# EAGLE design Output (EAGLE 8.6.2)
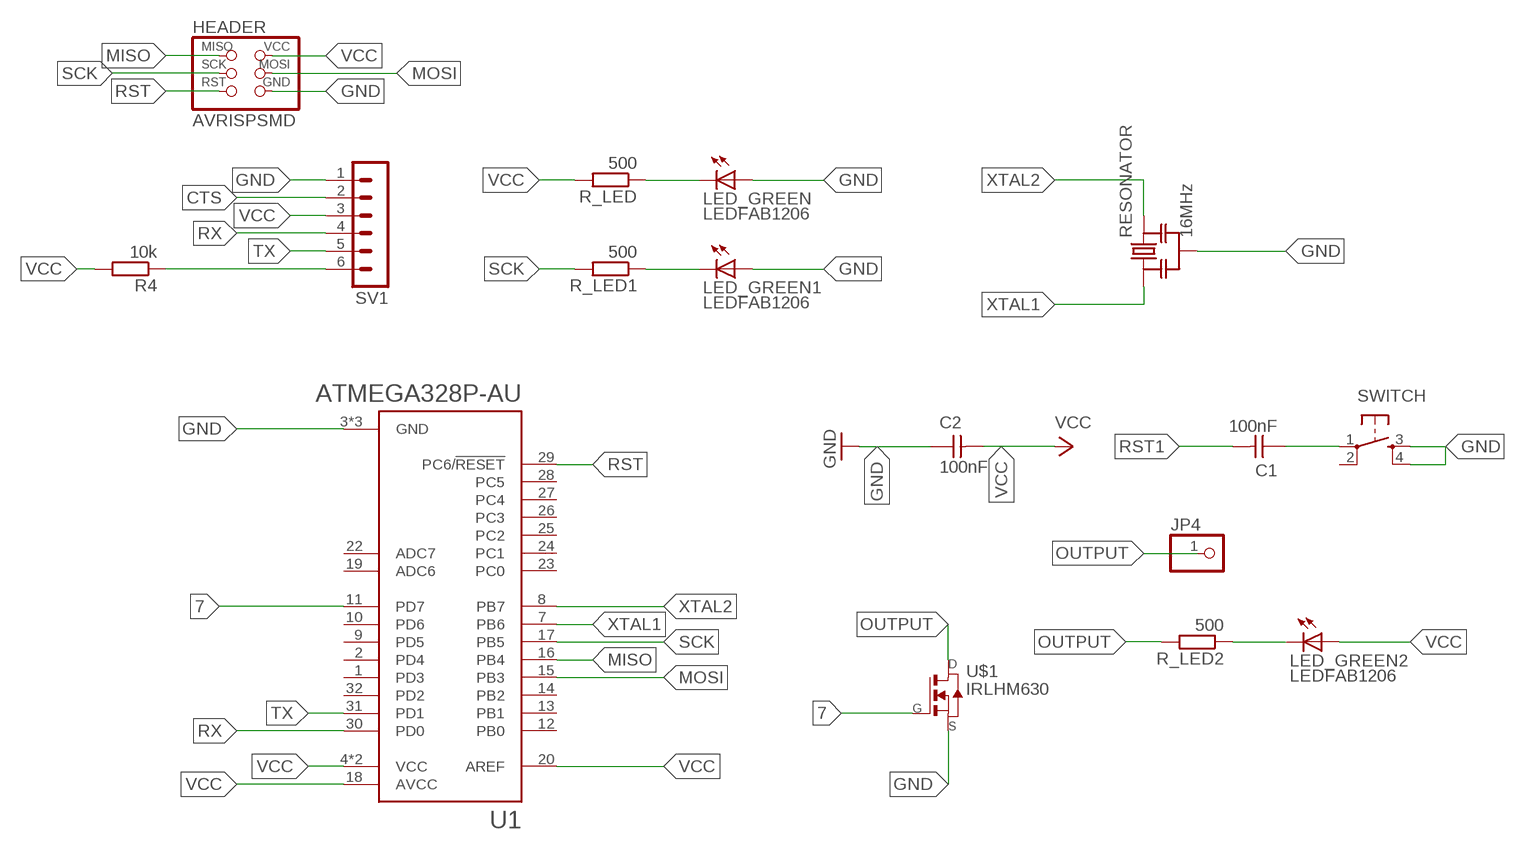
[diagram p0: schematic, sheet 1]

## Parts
C1  100nF  CAP-UNPOLARIZEDFAB  [C1206FAB]
C2  100nF  CAP-UNPOLARIZEDFAB  [C1206FAB]
HEADER  AVRISPSMD  [2X03SMD]
JP4  PINHD-1X1  [1X01]
LED_GREEN  LEDFAB1206  [LED1206FAB]
LED_GREEN1  LEDFAB1206  [LED1206FAB]
LED_GREEN2  LEDFAB1206  [LED1206FAB]
R4  10k  R-EU_R1206  [R1206]
R_LED  500  R-EU_R1206  [R1206]
R_LED1  500  R-EU_R1206  [R1206]
R_LED2  500  R-EU_R1206  [R1206]
RESONATOR  16MHz  RESONATOR-MURATACSTCR_G  [RESONATOR_MURATA3]
SV1  MA06-1  [MA06-1]
SWITCH  6MM_SWITCH6MM_SWITCH  [6MM_SWITCH]
U1  ATMEGA328P-AU  [QFP80P900X900X120-32N]
U$1  IRLHM630  [IRF-PQFN3.3X3.3B]

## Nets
7: U1.11(PD7) U$1.G
CTS: SV1.2
GND: C2.1 HEADER.6(GND) LED_GREEN1.1(A) LED_GREEN.1(A) RESONATOR.2 SV1.1 SWITCH.3(S) SWITCH.4(S1) U1.3(GND) U1.5(GND) U1.21(GND) U$1.S
MISO: HEADER.1(MISO) U1.16(PB4)
MOSI: HEADER.4(MOSI) U1.15(PB3)
N$1: LED_GREEN1.2(C) R_LED1.1
N$2: LED_GREEN2.2(C) R_LED2.1
N$21: LED_GREEN.2(C) R_LED.1
OUTPUT: JP4.1 R_LED2.2 U$1.D
RST: C1.1 HEADER.5(RST) SWITCH.1(P) U1.29(PC6/!RESET)
RST1: C1.2 R4.1 SV1.6
RX: SV1.4 U1.30(PD0)
SCK: HEADER.3(SCK) R_LED1.2 U1.17(PB5)
TX: SV1.5 U1.31(PD1)
VCC: C2.2 HEADER.2(VCC) LED_GREEN2.1(A) R4.2 R_LED.2 SV1.3 U1.4(VCC) U1.6(VCC) U1.18(AVCC) U1.20(AREF)
XTAL1: RESONATOR.1 U1.7(PB6)
XTAL2: RESONATOR.3 U1.8(PB7)
Unconnected: SWITCH.2(P1) U1.1(PD3) U1.2(PD4) U1.9(PD5) U1.10(PD6) U1.12(PB0) U1.13(PB1) U1.14(PB2) U1.19(ADC6) U1.22(ADC7) U1.23(PC0) U1.24(PC1) U1.25(PC2) U1.26(PC3) U1.27(PC4) U1.28(PC5) U1.32(PD2)

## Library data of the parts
C1 C2 = fab:CAP-UNPOLARIZED
HEADER = fab:AVRISP
JP4 = pinhead:PINHD-1X1: PIN HEADER
LED_GREEN LED_GREEN1 LED_GREEN2 = fab:LED: LED
R4 R_LED R_LED1 R_LED2 = resistor:R-EU_: RESISTOR, European symbol
RESONATOR = m-pad-2.1:RESONATOR-MURATA: Murata ceramic Resonator "ceralock" CSTCE series with built in load capacitance +- 0.5% tolerance 12.51MHz to 19.99MHz 16MHz murata part#: CSTCE16M0V53-R0 16MHz digikey part#: 490-1198-1-ND $1.33 each
SV1 = con-lstb:MA06-1: PIN HEADER; OC_FARNELL: unknown; OC_NEWARK: unknown
SWITCH = fab:6MM_SWITCH: OMRON SWITCH
U1 = ATMEGA328P-AU:ATMEGA328P-AU: ATmega Series 20 MHz 32 KB Flash 2 KB SRAM 8-Bit Microcontroller - TQFP-32; AVAILABILITY: Good; DESCRIPTION: ATmega Series 20 MHz 32 KB Flash 2 KB SRAM 8-Bit Microcontroller - TQFP-32; MF: Atmel; MP: ATMEGA328P-AU; PACKAGE: TQFP-32 Atmel; PRICE: 2.38 USD
U$1 = fab:IRLHM630

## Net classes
0 default: clearance 0.205 mm

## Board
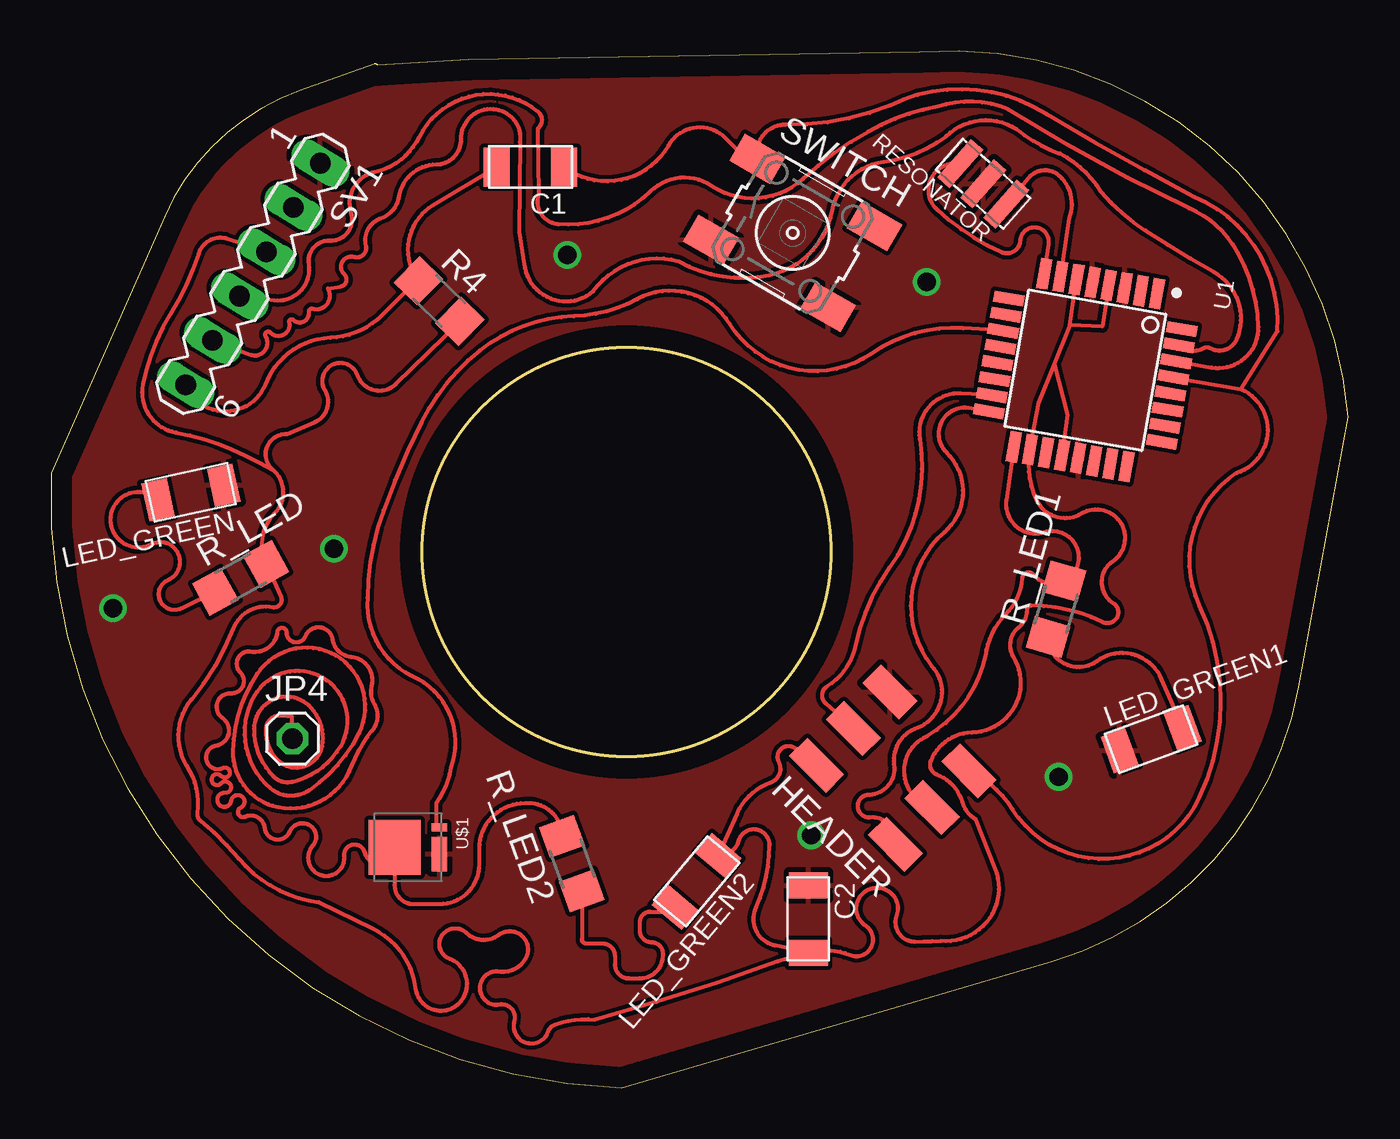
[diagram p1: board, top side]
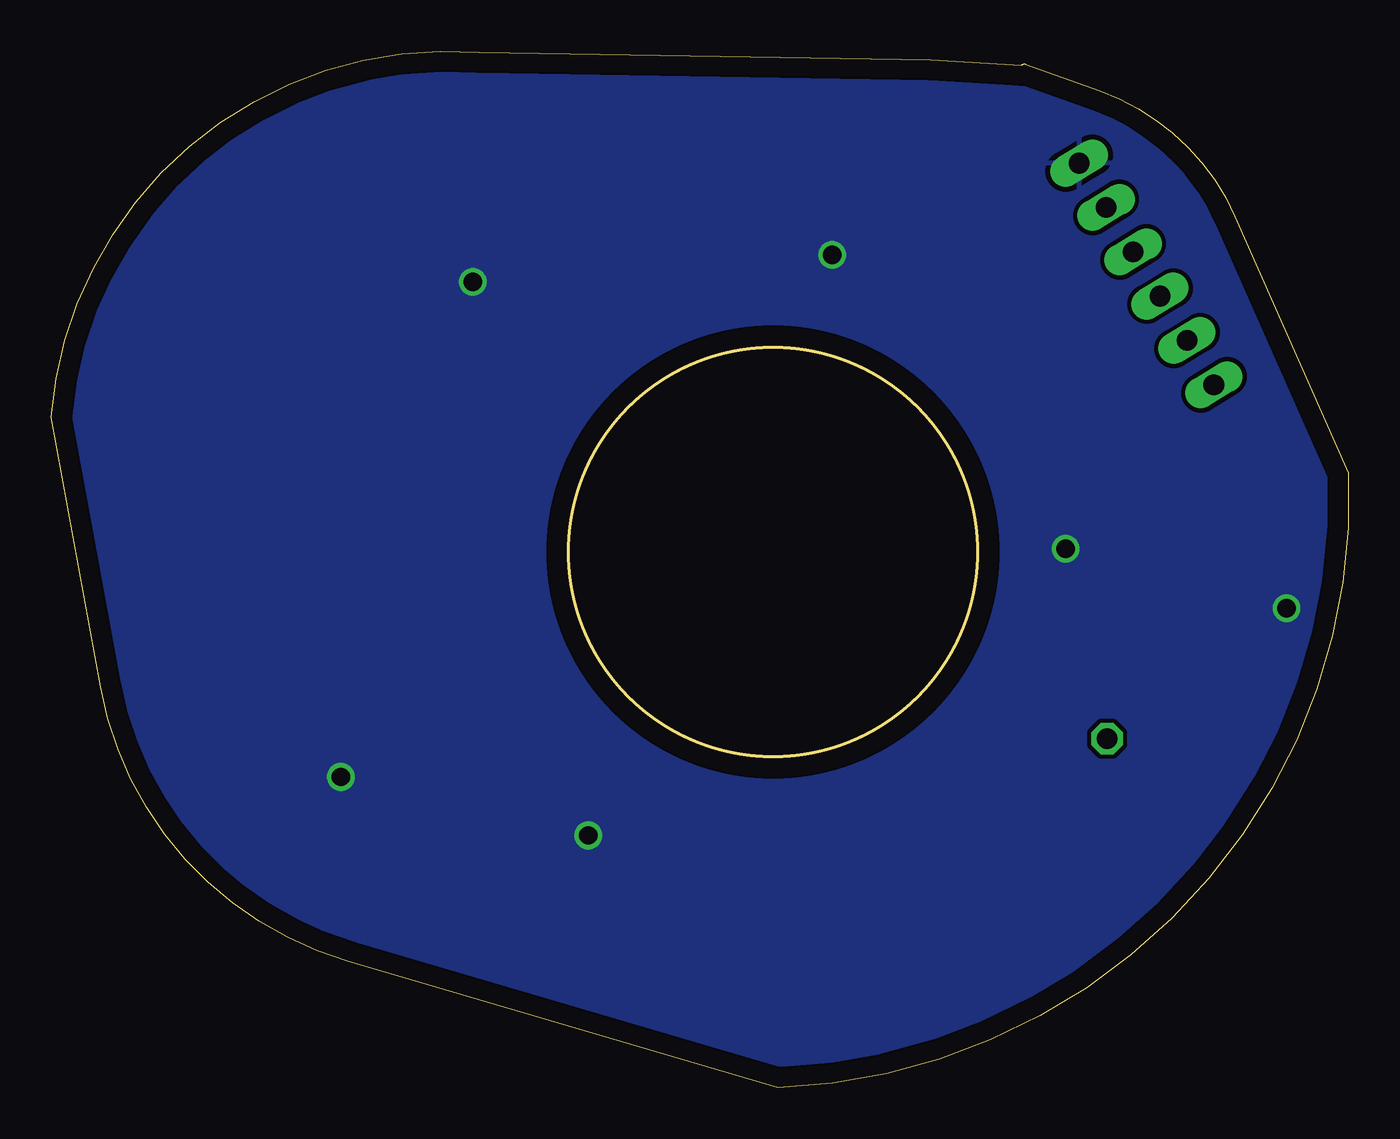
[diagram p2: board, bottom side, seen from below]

Size 63.52 x 50.75 mm. Coordinates in mm from the lower left corner, seen from the top.
Outline: 16,50.07 arc65 15.81,50.11 12.16,48.8 arc46 5.56,42.65 0,30.09 arc90 27.94,0 49,6.18 arc63 61.1,19.61 63.52,32.82 arc90 42.53,50.7 20.45,50.32 16,50.07
Outline: circle at 28.17,26.22 radius 10
Copper layers (1*16): Top 0.035mm / dielectric 1.5mm / Bottom 0.035mm
Design rules "default *": minimum track width 6mil, minimum drill 0.35mm, track to track 8mil, track to pad 8mil, pad to pad 8mil, via to via 8mil, smd to smd 8mil, copper to edge 40mil, drill to drill 8mil, minimum pad ring 10mil, minimum via ring 8mil, stop-mask expansion 4mil, vias tented up to drill 0mil, thermal gap 10mil

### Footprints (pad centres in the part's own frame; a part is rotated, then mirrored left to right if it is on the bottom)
C1206FAB = smd 1.27 x 1.905: 1 -1.651,0; 2 1.651,0
2X03SMD = smd 2.54 x 1.27: 1 -2.54,2.54; 2 2.92,2.54; 3 -2.54,0; 4 2.92,0; 5 -2.54,-2.54; 6 2.92,-2.54
1X01 = drill 1.016 octagon: 1 0,0
LED1206FAB = smd 1.27 x 1.905: 1 -1.651,0; 2 1.651,0
R1206 = smd 1.6 x 1.803: 1 -1.422,0; 2 1.422,0
RESONATOR_MURATA3 = smd 0.8 x 2.5: 1 -1.5,0; 2 0,0; 3 1.5,0
MA06-1 = drill 1.016 long: 1 -6.35,0; 2 -3.81,0; 3 -1.27,0; 4 1.27,0; 5 3.81,0; 6 6.35,0
6MM_SWITCH = smd 2.286 x 1.524: 1 -3.302,2.286; 2 3.302,2.286; 3 -3.302,-2.286; 4 3.302,-2.286
QFP80P900X900X120-32N = smd 1.5 x 0.55: 1 -4.3,2.8; 2 -4.3,2; 3 -4.3,1.2; 4 -4.3,0.4; 5 -4.3,-0.4; 6 -4.3,-1.2; 7 -4.3,-2; 8 -4.3,-2.8; 17 4.3,-2.8; 18 4.3,-2; 19 4.3,-1.2; 20 4.3,-0.4; 21 4.3,0.4; 22 4.3,1.2; 23 4.3,2; 24 4.3,2.8 | smd 0.55 x 1.5: 9 -2.8,-4.3; 10 -2,-4.3; 11 -1.2,-4.3; 12 -0.4,-4.3; 13 0.4,-4.3; 14 1.2,-4.3; 15 2,-4.3; 16 2.8,-4.3; 25 2.8,4.3; 26 2,4.3; 27 1.2,4.3; 28 0.4,4.3; 29 -0.4,4.3; 30 -1.2,4.3; 31 -2,4.3; 32 -2.8,4.3
IRF-PQFN3.3X3.3B = smd 2.7 x 2.54: D 0,-1.27 | smd 0.39 x 0.77: G -0.975,0.925 | smd 1.69 x 0.77: S 0.325,0.925

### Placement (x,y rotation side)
C1  23.47,45.07 180 top
C2  37.08,8.25 270 top
HEADER  41.35,15.51 135 top
JP4  11.82,17.08 0 top
LED_GREEN  6.85,29.14 192.4 top
LED_GREEN1  53.86,17.06 20 top
LED_GREEN2  31.61,10.09 230 top
R4  19,38.51 315.6 top
R_LED  9.28,24.96 28.9 top
R_LED1  49.21,23.43 74 top
R_LED2  25.5,10.96 110 top
RESONATOR  45.64,44.25 138.6 top
SV1  9.89,39.84 238.7 top
SWITCH  36.31,41.85 330 top
U1  50.64,35.13 260 top
U$1  18.09,11.76 270 top

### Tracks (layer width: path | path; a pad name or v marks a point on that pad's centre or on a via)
7
  Top 0.2: U1.11 44.66,37.18 arc38 40.16,35.93 arc-93 33.23,37.39 arc87 28.7,38.61 arc-26 25.59,37.77 arc36 21,36.09 arc25 18.14,32.58 arc6 16.28,28.26 arc20 15.5,23.98 arc69 17.67,20.16 arc-86 19.57,15.65 arc-26 18.85,13.91 18.85,12.74 U$1.G
GND  (via drill 0.9)
  other vias: 13.86,26.39 49.34,15.21 37.23,12.35 42.87,39.44 25.27,40.78 3.03,23.46
  pour Top: -37.68,78.67 -0.24,-8.88 7.37,-16.26 75.76,-78.44 85.51,-52.14 85.51,79.94 75.35,90.1 -26.25,90.1
  pour Bottom: -11.95,28.08 1.62,41.65 1.62,52.26 8.59,59.22 28.17,59.22 51.51,59.22 62.64,48.09 67.98,42.75 67.98,26.02 67.98,11.04 53.51,-3.43 17.72,-3.43 15.19,-0.9 -4.71,19 -8.78,19 -8.78,24.7 -12,27.92
MISO
  Top 0.2: U1.16 44.93,33.27 arc145 43.84,31.1 arc-95 43.74,27.19 arc87 43.12,20.64 arc-111 42.43,17.62 arc84 41.29,15.67 arc-93 39.96,14.33 arc177 40.09,13.24 arc-103 HEADER.1
MOSI
  Top 0.2: U1.15 44.54,33.99 arc102 42.53,31.76 arc-44 41.06,25.47 arc24 39.39,21.64 arc-46 37.99,19.63 arc106 37.91,18.82 arc0 HEADER.4
N$1
  Top 0.2: LED_GREEN1.2 54.37,20.01 arc102 51.19,20.87 arc-125 R_LED1.1
N$2
  Top 0.2: R_LED2.1 25.99,7.26 arc90 26.2,7.06 27,7.06 arc-90 27.6,6.45 27.6,6.03 arc90 28.28,5.35 28.83,5.35 arc90 29.96,6.48 29.96,6.55 arc90 29.41,7.11 | 29.41,7.11 | 29.41,7.11 arc-90 28.83,7.68 28.83,8.11 arc-90 29.34,8.61 30.33,8.61 arc90 LED_GREEN2.2
N$21
  Top 0.2: R_LED.1 6.39,23.46 arc-182 5.74,24.86 arc184 4.91,26.59 arc-252 LED_GREEN.2
OUTPUT
  Top 0.2: JP4.1 11.8,18.16 11.25,18.21 arc90 10.53,17.61 arc51 11.1,16.03 arc124 13.27,16.71 arc59 12.6,18.73 arc131 9.93,17.56 arc46 10.89,15.23 arc57 11.8,14.97 arc47 14.18,16.71 arc180 9.96,19.19 arc80 10.74,14.66 arc74 12.63,14.56 arc30 15.08,17.35 arc173 10.09,20.25 arc32 8.9,16.5 arc81 11.12,13.73 arc80 14.72,15.75 arc-19 15.73,17.48 arc71 15.84,18.78 arc-45 15.71,19.66 arc99 14.7,21.08 arc-76 13.79,21.93 arc150 12.44,22.09 arc-159 11.54,22.27 arc175 11.07,22.3 arc-42 10.74,21.62 arc-52 9.78,21.34 arc144 9.26,20.33 arc-138 8.8,19.29 arc149 8.38,18.1 arc-136 8.07,16.73 arc196 8.41,15.65 arc-253 8.33,15.26 arc275 8.33,14.89 arc-233 8.51,14.43 arc268 8.82,14.04 arc-237 9.29,13.7 arc179 9.49,13.26 arc-108 10.45,12.72 arc151 11.69,12.54 arc-198 12.81,11.84 arc228 14.36,11.35 arc-172 15.34,11.53 arc169 U$1.D 16.82,9.9 arc90 17.73,8.99 19.04,8.99 arc90 20.97,10.92 20.97,11.7 arc-90 23.21,13.93 23.38,13.93 arc-90 R_LED2.2
RST
  Top 0.2: 58.25,34.21 arc-138 58.04,30.09 arc82 56.21,23.64 arc-50 56.21,14.18 arc-123 47.08,13.63 arc33 HEADER.5 | U1.29 58.25,34.21 | 58.25,34.21 60.05,37.03 arc71 55.98,43.61 arc-3 48.76,47.65 arc58 41.06,48.09 arc-23 35.95,47.14 arc104 SWITCH.1 34.03,45.48 33.02,46.49 arc105 30.22,46.12 arc-97 C1.1
RST1
  Top 0.2: C1.2 18.7,43.2 arc96 R4.1 17.89,39.51 16.21,37.83 arc-43 13.67,36.71 arc66 10.5,34.44 arc-137 SV1.6
RX
  Top 0.2: SV1.4 10.94,38.55 arc106 12.63,40.31 arc-102 13.66,41.48 arc110 14.7,42.82 arc-95 15.86,44.84 arc51 18.04,46.55 arc-103 23.83,47.79 arc-101 23.83,46.96 23.89,43.72 arc104 24.83,42.27 arc49 29.35,43.88 arc-78 32.35,44.15 arc77 36.82,44.5 arc-14 40.02,46.81 arc-18 43.41,48.03 arc-40 46.86,47.91 arc7 55.73,43.05 arc-33 57.83,41.32 arc-33 59.12,37.24 arc-101 56.82,35.26 U1.30
SCK
  Top 0.2: U1.17 46.77,28.76 arc116 48.62,27.19 arc-171 R_LED1.2 arc-77 48.1,25.11 arc136 47.55,24.93 arc-41 46.74,23.17 arc38 45.75,21.16 arc-48 42.89,17.2 arc142 HEADER.3
TX
  Top 0.2: SV1.5 9.75,35.89 arc142 10.5,36.79 arc-167 10.74,36.97 arc149 11.67,37.49 arc-148 11.85,37.59 arc142 12.63,37.98 arc-114 12.81,38.14 arc138 13.56,39.12 14.18,39.22 arc127 14.36,39.82 arc-153 14.85,40.67 arc120 15.42,41.22 arc-84 16.15,42.56 arc61 17.05,43.65 arc-81 18.86,45.2 arc91 20.08,46.44 arc-129 22.44,47.61 arc-60 22.96,46.31 22.92,41.92 23.17,40.31 arc124 26.54,38.99 arc-70 30.73,40.46 arc41 35.16,39.78 arc68 38.25,42.94 arc-72 40.78,45.33 arc29 43.83,46.59 arc-77 47.28,46.92 arc21 49.4,45.74 arc-31 51.4,43.87 arc16 53.58,41.96 arc4 56.91,39.95 arc-84 58.03,36.62 arc-96 56.76,36.2 arc60 56.42,36.2 arc-74 U1.31
VCC
  Top 0.2: 49.11,35.39 48.36,33.54 U1.18 arc36 48.25,28.78 arc96 50.46,28.11 arc-177 51.97,25.76 arc114 52,23.73 arc-174 51.48,22.79 arc26 48,23.6 arc90 47.78,23.38 arc-51 47.37,22.52 arc82 47.11,21.08 arc-120 45.08,17.38 arc67 43.07,16 arc91 43.36,15.33 arc-53 44.62,13.97 arc43 45.26,13.14 46.22,10.7 arc-117 43.56,7.18 arc-4 42.29,7.15 arc-110 41.4,8.43 arc256 39.88,7.92 arc-169 39.13,6.49 arc38 C2.2 | 49.11,35.39 49.89,37.3 49.89,37.32 | 49.89,37.32 U1.6 | U1.4 51.47,37.27 49.89,37.32 | 49.11,35.39 49.77,32.93 U1.20 | 10.87,30.24 arc-94 10.97,28.15 arc68 R_LED.2 11.25,24.03 arc-126 10.84,23.51 arc80 8.92,22.48 arc-18 6.85,18.98 arc72 6.65,15.75 arc-39 7.16,13.45 arc58 7.32,13.06 arc-10 9.18,11.22 arc42 13.12,9.07 15.75,7.78 arc-57 17.84,4.87 arc128 19.99,4.14 arc114 19.52,6.3 arc-203 20.32,7.58 arc80 21.93,7.48 arc-152 23.26,6.38 arc-73 21.93,5.67 arc199 21.95,4.07 arc-116 22.68,3.26 arc176 24.34,2.74 arc-51 24.69,3.09 arc-25 26.63,3.33 arc5 35.58,6.17 C2.2 | 10.87,30.24 arc-143 11.56,32 12.93,32.59 arc104 13.35,34.23 arc-185 15.01,34.88 arc115 16.87,34.44 R4.2 | SV1.3 8.64,41.55 arc91 7.22,40.83 arc-14 5.84,37.85 arc21 4.5,34.41 arc91 6.1,32.08 arc-14 8.82,31.25 arc-5 10.87,30.24 | LED_GREEN2.1 | LED_GREEN2.1 33.6,13.43 arc-47 35.23,14.93 arc98 35.64,15.95 arc-189 36.6,16.37 arc75 HEADER.2 | C2.2 35.44,6.95 arc-102 34.52,8.8 arc24 35.18,11.87 arc165 33.66,12.07 arc-79 LED_GREEN2.1
XTAL1
  Top 0.2: RESONATOR.1 47.88,44.56 arc-93 49.37,44.65 arc-69 49.84,42.55 U1.7
XTAL2
  Top 0.2: U1.8 48.85,41.31 arc185 47.44,41.45 arc-110 46.54,40.9 arc-19 43.39,42.98 arc-147 RESONATOR.3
